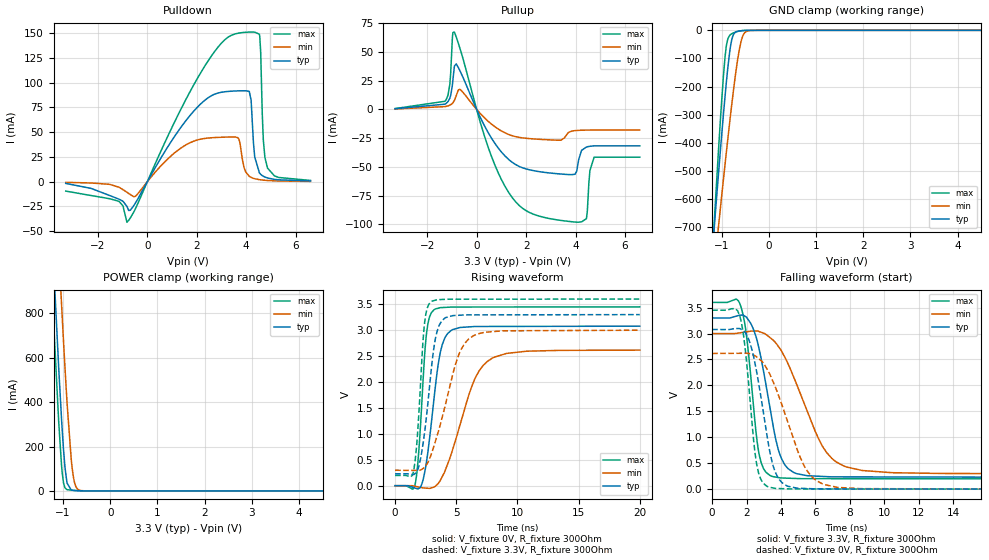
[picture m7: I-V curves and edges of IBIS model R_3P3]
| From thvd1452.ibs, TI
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|   R_3P3 Model
[Model]   R_3P3
Model_type   3-state
Polarity   Non-Inverting
Vmeas = 1.65
Vref = 0
Cref = 15pF
Rref = 100000
|   typ   min   max
C_comp   7.272pF   7.106pF   7.475pF
|  Where Nom  PVT is Nominal Process,   3.3V,  25C
|   Fast PVT is Strong Process,   3.6V, -40C
|   Slow PVT is Weak Process,   3V, 150C
[Voltage Range]   3.3   3   3.6
|Junction Temperature
[Temperature Range]   25   150   -40
[Pullup Reference]   3.3   3   3.6
[Pulldown Reference]   0   0   -0
[Power Clamp Reference]   3.3   3   3.6
[GND Clamp Reference]   0   0   0
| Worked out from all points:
|   slope of the pulldown table from 0 to 0.495 V, typ, clamps not added: 22.9 ohm
|   slope of the pullup table from 0 to 0.495 V, typ, clamps not added: 23.3 ohm
|   GND clamp passes 1 mA (typ) near -0.56 V on its own axis
|   POWER clamp passes 1 mA (typ) near -0.67 V on its own axis
|   falling waveform, V_fixture 3.3V, R_fixture 300Ohm: 20-80 % time 1.04ns typ, 2.04ns min, 619ps max; typ from 3.3 V to 0.23 V
|   rising waveform, V_fixture 0V, R_fixture 300Ohm: 20-80 % time 951ps typ, 2.12ns min, 551ps max; typ from 0 V to 3.08 V
|   rising waveform, V_fixture 3.3V, R_fixture 300Ohm: 20-80 % time 883ps typ, 1.83ns min, 528ps max; typ from 0.23 V to 3.3 V
|   falling waveform, V_fixture 0V, R_fixture 300Ohm: 20-80 % time 953ps typ, 1.73ns min, 594ps max; typ from 3.08 V to 0 V
[Pulldown]
|   Voltage   I(typ)   I(min)   I(max)
-3.3V     -1.729mA   -655.1uA   -9.49mA
-1.147V   -17.66mA   -5.603mA   -19.81mA
-824.9mV  -24.97mA   -10.66mA   -40.91mA
2.339V    82.53mA    43.75mA    117.4mA
3.666V    91.77mA    44.44mA    150mA
4.123V    91.25mA    5.492mA    151.2mA
4.2V      82.07mA    4.323mA    151.1mA
4.344V    25.07mA    3.001mA    151.1mA
4.549V    8.499mA    2.003mA    147mA
4.694V    5.479mA    1.577mA    41.97mA
4.862V    3.775mA    1.232mA    13.8mA
6.6V      725.2uA    297.7uA    1.276mA
[GND Clamp]
|   Voltage   I(typ)   I(min)   I(max)
-3.3V     -5.574A    -4.524A    -7.37A
-1.176V   -743.8mA   -877.1mA   -741.4mA
-1.125V   -633.4mA   -792.5mA   -591.8mA
-1.063V   -504.9mA   -693.2mA   -420.1mA
-926.2mV  -232.9mA   -475.2mA   -93.33mA
-895.8mV  -178.7mA   -428.3mA   -51.39mA
-824.9mV  -72.33mA   -321.6mA   -17.07mA
-731.1mV  -10.51mA   -190mA     -7.947mA
-662mV    -3.564mA   -106mA     -4.061mA
-568.5mV  -1.111mA   -28.27mA   -1.242mA
-400.8mV  -67.49uA   -653.7uA   -47.19uA
6.6V      0A         0A         0A
[Pullup]
|   Voltage   I(typ)   I(min)   I(max)
-3.3V     560.1uA    370.5uA    728.3uA
-1.278V   4.569mA    2.429mA    7.078mA
-1.085V   9.719mA    3.69mA     21.67mA
-899.7mV  37.67mA    7.766mA    67.27mA
588.8mV   -24.59mA   -12.6mA    -40.21mA
1.861V    -50.84mA   -24.8mA    -86.1mA
3.982V    -56.41mA   -18.45mA   -98.02mA
4.244V    -35.68mA   -18.11mA   -97.86mA
4.442V    -32.74mA   -18.02mA   -95.02mA
4.585V    -32.09mA   -17.98mA   -53.08mA
4.754V    -31.72mA   -17.96mA   -41.54mA
6.6V      -31.72mA   -17.96mA   -41.54mA
[POWER Clamp]
|   Voltage   I(typ)   I(min)   I(max)
-3.3V     11.22A     11.71A     11A
-1.249V   1.241A     1.795A     985.5mA
-1.198V   1.016A     1.569A     760.7mA
-1.09V    553.2mA    1.093A     310.5mA
-1.032V   328.7mA    847.9mA    118.7mA
-987.6mV  184.1mA    670.5mA    34.96mA
-917.6mV  39.86mA    410.4mA    6.101mA
-824.9mV  3.812mA    142mA      3.29mA
-784.8mV  2.338mA    70.64mA    2.65mA
-719.5mV  1.432mA    16.69mA    1.743mA
-629.9mV  696.7uA    2.159mA    783.2uA
6.6V      0A         0A         0A
[Ramp]
R_load = 300
|   typ   min   max
dV/dt_r   1.84616/9.47025e-10   1.56867/2.11704e-09   2.06964/5.49202e-10
dV/dt_f   1.84214/1.03769e-09   1.62061/2.04134e-09   2.04095/6.18768e-10
[Falling Waveform]
V_fixture = 3.3V
V_fixture_min = 3V
V_fixture_max = 3.6V
R_fixture = 300Ohm
C_fixture = 0F
|   Time   V(typ)   V(min)   V(max)
0s        3.3V       2.999V     3.6V
1.66ns    3.354V     3.015V     3.527V
2.011ns   3.306V     3.033V     2.916V
2.7ns     2.741V     3.041V     725.1mV
3.363ns   1.561V     2.92V      263.3mV
3.865ns   738.8mV    2.743V     222.7mV
4.41ns    395.4mV    2.415V     211.4mV
6.35ns    246.5mV    862.6mV    202.3mV
7.629ns   237.1mV    450.3mV    201.9mV
20ns      229.6mV    298.3mV    198.4mV
[Rising Waveform]
V_fixture = 0V
V_fixture_min = 0V
V_fixture_max = 0V
R_fixture = 300Ohm
C_fixture = 0F
|   Time   V(typ)   V(min)   V(max)
0s        266.4uV    702.8uV    62.26uV
1.638ns   -44.93mV   -10.88mV   25.31mV
1.942ns   -52.48mV   -25.47mV   674.8mV
2.548ns   430.2mV    -46.59mV   2.888V
3.175ns   1.662V     -26.29mV   3.392V
3.704ns   2.578V     105.8mV    3.435V
4.28ns    2.93V      406.6mV    3.442V
6.471ns   3.07V      2.034V     3.447V
7.918ns   3.072V     2.456V     3.447V
20ns      3.077V     2.615V     3.449V
[Rising Waveform]
V_fixture = 3.3V
V_fixture_min = 3V
V_fixture_max = 3.6V
R_fixture = 300Ohm
C_fixture = 0F
|   Time   V(typ)   V(min)   V(max)
0s        229.6mV    298.3mV    198.4mV
1.496ns   213.8mV    294.8mV    263mV
1.837ns   300.7mV    294mV      1.003V
2.389ns   985.7mV    356.7mV    3.089V
2.942ns   2.202V     597.7mV    3.55V
3.325ns   2.868V     879.5mV    3.581V
3.803ns   3.174V     1.276V     3.592V
5.173ns   3.287V     2.505V     3.597V
6.35ns    3.295V     2.885V     3.598V
20ns      3.3V       2.999V     3.6V
[Falling Waveform]
|Gnd
V_fixture = 0V
V_fixture_min = 0V
V_fixture_max = 0V
R_fixture = 300Ohm
C_fixture = 0F
|   Time   V(typ)   V(min)   V(max)
0s        3.077V     2.615V     3.449V
1.592ns   3.095V     2.619V     3.349V
1.925ns   3.014V     2.62V      2.691V
2.568ns   2.29V      2.553V     517.6mV
3.175ns   1.059V     2.322V     56.64mV
3.554ns   437.2mV    2.06V      22.68mV
4.059ns   124.3mV    1.619V     9.922mV
5.313ns   14.91mV    471.6mV    3.698mV
6.413ns   5.424mV    101.2mV    3.426mV
20ns      266.3uV    702.7uV    61.95uV
